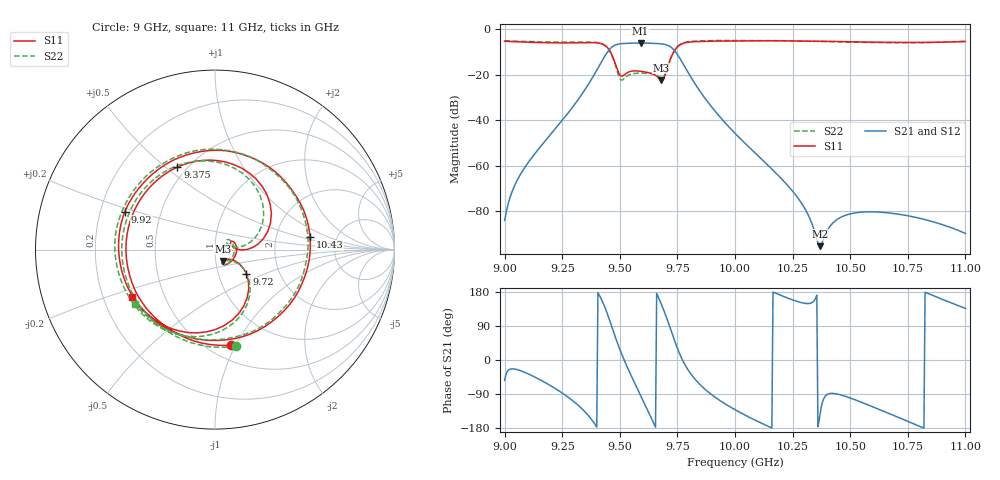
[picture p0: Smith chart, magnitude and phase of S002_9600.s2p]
# Hz S DB R 50
! Planar, S50180, , 20.4.1/1
! Date: 14.11.2021 18:36:07
! Data: Format (Calibration Info)
! Freq	S11:dB/Ang(--)	S21:dB/Ang(--)	S12:dB/Ang(--)	S22:dB/Ang(--)
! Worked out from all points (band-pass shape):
!   401 points, 9 GHz to 11 GHz, reference 50 ohm
!   highest |S21| = -6.14 dB at 9.59 GHz (marker M1); lowest = -95.5 dB at 10.37 GHz (marker M2)
!   |S21| within 3 dB of the highest: 9.454 GHz to 9.735 GHz (280.9 MHz wide, 2.93 % of centre)
!   lowest |S11| = -22.4 dB at 9.68 GHz (marker M3), VSWR 1.16, Z = 54 - j6.83 ohm
!   |S11| at or under -10 dB: 9.459 GHz to 9.734 GHz (275 MHz wide, 2.87 % of centre)
!   |S22| runs from -22.4 to -5.0 dB; largest |S21 - S12| = 0.00053
!   S11 on the Smith chart (normalised r, x): 9 GHz: 0.64, -0.96; 9.375 GHz: 0.44, +0.55; 9.72 GHz: 1.36, -0.39; 9.92 GHz: 0.31, +0.18; 10.43 GHz: 3.16, +0.62; 11 GHz: 0.32, -0.24
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9e9  -5.35 -80.6  -84.11 -53.9  -84.12 -53.9  -5.17 -78.0
9.09e9  -5.74 -110.5  -60.48 -33.2  -60.48 -33.3  -5.45 -106.8
9.23e9  -6.08 -165.0  -42.63 -79.2  -42.64 -79.2  -5.68 -157.9
9.335e9  -5.99 141.8  -28.71 -128.3  -28.71 -128.3  -5.68 151.5
9.375e9  -5.93 114.5  -22.42 -155.2  -22.43 -155.2  -5.72 124.9
9.44e9  -7.51 46.5  -11.08 131.8  -11.09 131.7  -7.64 56.9
9.475e9  -13.57 3.2  -7.29 70.2  -7.29 70.2  -14.10 11.3
9.525e9  -19.70 26.6  -6.29 -8.4  -6.30 -8.5  -21.21 39.2
9.59e9  -18.56 -15.9  -6.14 -93.4  -6.15 -93.5  -19.41 -8.4
9.67e9  -21.61 -62.7  -6.41 162.0  -6.42 161.9  -20.95 -61.5
9.68e9  -22.38 -55.6  -6.50 147.6  -6.50 147.6  -21.54 -56.3
9.72e9  -13.10 -37.8  -7.79 82.3  -7.79 82.3  -13.04 -37.4
9.78e9  -6.12 -113.0  -16.21 -9.4  -16.21 -9.4  -5.91 -107.4
9.84e9  -5.50 -161.4  -26.14 -59.8  -26.14 -59.8  -5.23 -153.0
9.92e9  -5.28 157.3  -36.89 -101.0  -36.89 -101.0  -5.02 168.4
1e10  -5.24 126.8  -45.82 -131.1  -45.83 -131.1  -5.03 139.4
1.0155e10  -5.14 79.3  -61.05 -177.9  -61.05 -177.9  -5.03 92.9
1.0335e10  -5.34 30.7  -85.81 151.8  -85.82 151.8  -5.37 43.6
1.037e10  -5.36 21.6  -95.45 -139.7  -95.46 -139.7  -5.42 34.2
1.0425e10  -5.45 7.5  -85.24 -88.1  -85.24 -88.1  -5.55 19.3
1.067e10  -5.84 -58.6  -80.87 -141.6  -80.87 -141.6  -5.99 -50.9
1.1e10  -5.48 -150.4  -89.87 136.1  -89.87 136.1  -5.37 -145.5
